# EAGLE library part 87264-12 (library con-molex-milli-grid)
RECEPTACAL
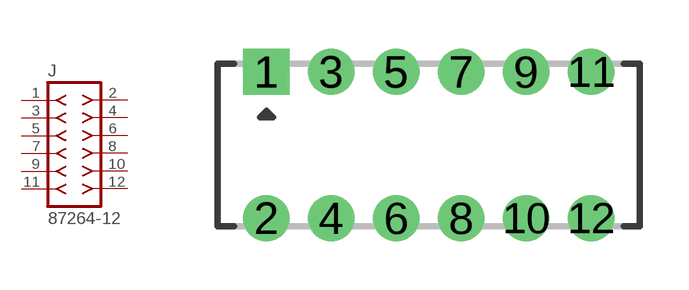
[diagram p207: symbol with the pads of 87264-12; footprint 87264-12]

Designator prefix J

## 87264-12  [87264-12]
1  1  pas
2  2  pas
3  3  pas
4  4  pas
5  5  pas
6  6  pas
7  7  pas
8  8  pas
9  9  pas
10  10  pas
11  11  pas
12  12  pas

## Footprint 87264-12 (pad centres in mm)
RECEPTACAL Dual Row, Side Entry
drill 0.914 square: 1 -5,2.25
drill 0.914: 2 -5,-2.25; 3 -3,2.25; 4 -3,-2.25; 5 -1,2.25; 6 -1,-2.25; 7 1,2.25; 8 1,-2.25; 9 3,2.25; 10 3,-2.25; 11 5,2.25; 12 5,-2.25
